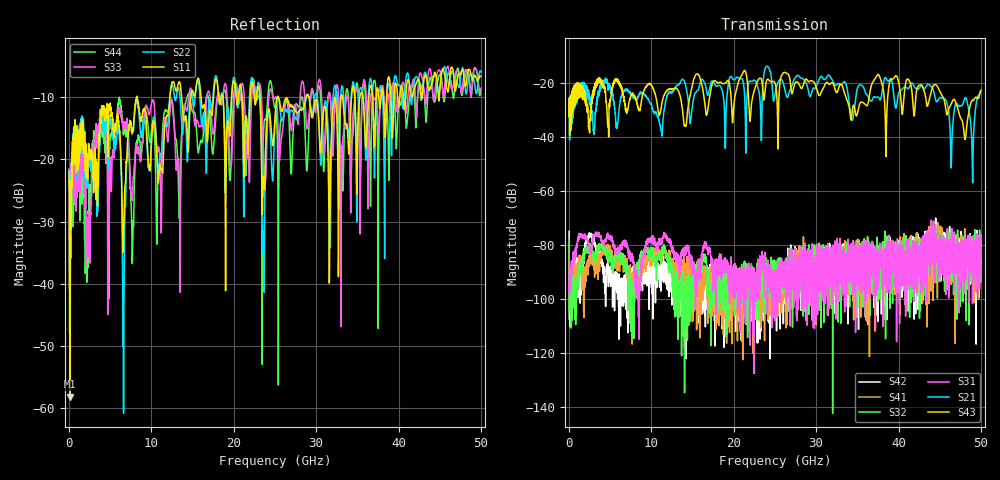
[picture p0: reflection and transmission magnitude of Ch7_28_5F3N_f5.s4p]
!Agilent Technologies,N5247A,US51170199,A.09.90.13
!Agilent N5247A: A.09.90.13
!Date: Wednesday, December 09, 2015 09:26:47
!Correction: S11(Full 4 Port(1,2,3,4))
!S12(Full 4 Port(1,2,3,4))
!S13(Full 4 Port(1,2,3,4))
!S14(Full 4 Port(1,2,3,4))
!S21(Full 4 Port(1,2,3,4))
!S22(Full 4 Port(1,2,3,4))
!S23(Full 4 Port(1,2,3,4))
!S24(Full 4 Port(1,2,3,4))
!S31(Full 4 Port(1,2,3,4))
!S32(Full 4 Port(1,2,3,4))
!S33(Full 4 Port(1,2,3,4))
!S34(Full 4 Port(1,2,3,4))
!S41(Full 4 Port(1,2,3,4))
!S42(Full 4 Port(1,2,3,4))
!S43(Full 4 Port(1,2,3,4))
!S44(Full 4 Port(1,2,3,4))
!S4P File: Measurements: <S11,S12,S13,S14>,
!<S21,S22,S23,S24>,
!<S31,S32,S33,S34>,
!<S41,S42,S43,S44>:
# Hz S  dB  R 50
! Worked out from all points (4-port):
!   3201 points, 10 MHz to 50 GHz, reference 50 ohm
!   strongest paths, dB at 10 MHz, 12.51 GHz, 25 GHz, 37.5 GHz, 50 GHz:
!     S43: -32.6, -22.5, -20.2, -17.0, -23.0
!     S21: -32.5, -23.5, -24.6, -25.3, -22.8
!     S31: -85.6, -80.7, -92.3, -96.3, -80.1
!     S32: -78.1, -88.0, -87.6, -101.0, -79.4
!     S41: -89.2, -88.7, -93.8, -91.0, -87.0
!     S42: -75.0, -93.8, -93.2, -87.4, -86.5
!   lowest |S11| = -58.1 dB at 135 MHz (marker M1), VSWR 1.00, Z = 50 + j0.12 ohm
!   |S11| at or under -10 dB: start of sweep to 8.234 GHz; 8.272 GHz to 12.25 GHz (3.983 GHz wide, 38.8 % of centre); 29.13 GHz to 33.03 GHz (3.901 GHz wide, 12.6 % of centre)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
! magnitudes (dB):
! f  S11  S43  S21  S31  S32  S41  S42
! 10 MHz  -22.0  -32.6  -32.5  -85.6  -78.1  -89.2  -75.0
! 135 MHz  -58.1  -35.1  -32.8  -92.6  -96.1  -96.2  -103.1
! 24.05 GHz  -13.1  -18.8  -14.0  -90.8  -87.0  -98.3  -101.4
! 34.36 GHz  -8.9  -31.0  -33.9  -94.9  -84.8  -86.8  -87.9
! 43.72 GHz  -8.8  -26.3  -20.8  -86.7  -79.1  -73.2  -78.8
! 48.97 GHz  -7.4  -26.6  -52.5  -81.6  -76.9  -82.4  -80.0
! 50 GHz  -6.6  -23.0  -22.8  -80.1  -79.4  -87.0  -86.5
